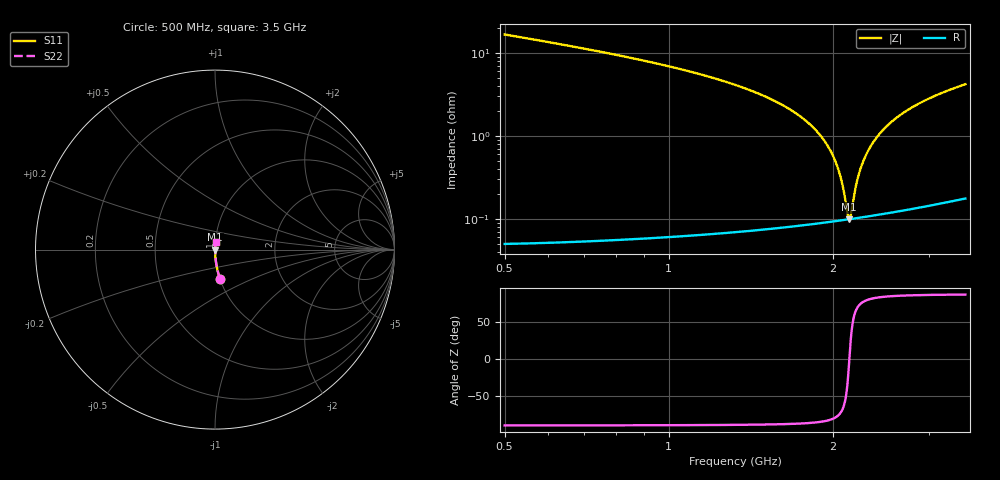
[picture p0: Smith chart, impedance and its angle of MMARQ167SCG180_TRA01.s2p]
! MMARQ167SCG180_TRA01  S-PARAMETER MODEL  ( General Type )
! Model Generated by TAIYO YUDEN Corporation (http://www.ty-top.com)
! Version 1.0
! TAIYO YUDEN Control No. 160201
! Copyright(c) 2016 TAIYO YUDEN CO.,LTD. All Rights Reserved.
! Product Description (link to TY-COMPAS)
! https://ds.yuden.co.jp/TYCOMPAS/or/detail?pn=MMARQ167SCG180JTRA01&u=M
! Products Name : Multilayer Ceramic Capacitors
! Characteristics :
!  Capacitance : 18 pF , Rated Voltage : 250V , TCC : CG / C0G
!  Case Size : 1.6 x 0.8 / 0.063 x 0.031 [mm/inch] , Thickness : 0.7 / 0.028 [mm/inch]
!  (Conditions: Temperature = 25 degC , DC Bias Current/Voltage = 0A / 0V)
! External Node Assignments :
!  1  o---| |---o  2
! GND o---------o GND
! Frequency Range : 500MHz  -  3500MHz  [ 401 STEP ]
# MHz S RI R 50
! Freq[MHz].  S11 Real  S11 Imag  S21 Real  S21 Imag  S12 Real  S12 Imag  S22 Real  S22 Imag
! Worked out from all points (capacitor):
!   401 points, 500 MHz to 3.5 GHz, reference 50 ohm
!   read as one part in series: C = 18 pF near 515 MHz
!   lowest |Z| = 99.2 mohm at 2.143 GHz (marker M1)
!   series resonance near 2.144 GHz, so ESL is about 310 pH
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500  0.0276 -0.1625  0.9724 0.1625  0.9724 0.1625  0.0276 -0.1625
1002.5  0.00531 -0.0685  0.9947 0.0685  0.9947 0.0685  0.00531 -0.0685
1505  0.00163 -0.0297  0.9984 0.0297  0.9984 0.0297  0.00163 -0.0297
1677.5  0.00122 -0.0204  0.9988 0.0204  0.9988 0.0204  0.00122 -0.0204
1812.5  0.00105 -0.0139  0.999 0.0139  0.999 0.0139  0.00105 -0.0139
1917.5  0.00098 -0.0092  0.999 0.0092  0.999 0.0092  0.00098 -0.0092
2000  0.000961 -0.00572  0.999 0.00572  0.999 0.00572  0.000961 -0.00572
2037.5  0.000962 -0.00419  0.999 0.00419  0.999 0.00419  0.000962 -0.00419
2067.5  0.000966 -0.00299  0.999 0.00299  0.999 0.00299  0.000966 -0.00299
2090  0.000971 -0.0021  0.999 0.0021  0.999 0.0021  0.000971 -0.0021
2127.5  0.000983 -0.000634  0.999 0.000634  0.999 0.000634  0.000983 -0.000634
2142.5  0.000989 -5.67e-05  0.999 5.67e-05  0.999 5.67e-05  0.000989 -5.67e-05
2157.5  0.000996 0.000517  0.999 -0.000517  0.999 -0.000517  0.000996 0.000517
2195  0.00102 0.00193  0.999 -0.00193  0.999 -0.00193  0.00102 0.00193
2217.5  0.00103 0.00277  0.999 -0.00277  0.999 -0.00277  0.00103 0.00277
2247.5  0.00105 0.00388  0.9989 -0.00388  0.9989 -0.00388  0.00105 0.00388
2277.5  0.00107 0.00497  0.9989 -0.00497  0.9989 -0.00497  0.00107 0.00497
2375  0.00117 0.00842  0.9988 -0.00842  0.9988 -0.00842  0.00117 0.00842
2502.5  0.00132 0.0128  0.9987 -0.0128  0.9987 -0.0128  0.00132 0.0128
2720  0.00166 0.0197  0.9983 -0.0197  0.9983 -0.0197  0.00166 0.0197
3005  0.00223 0.0282  0.9978 -0.0282  0.9978 -0.0282  0.00223 0.0282
3500  0.00351 0.0417  0.9965 -0.0417  0.9965 -0.0417  0.00351 0.0417
